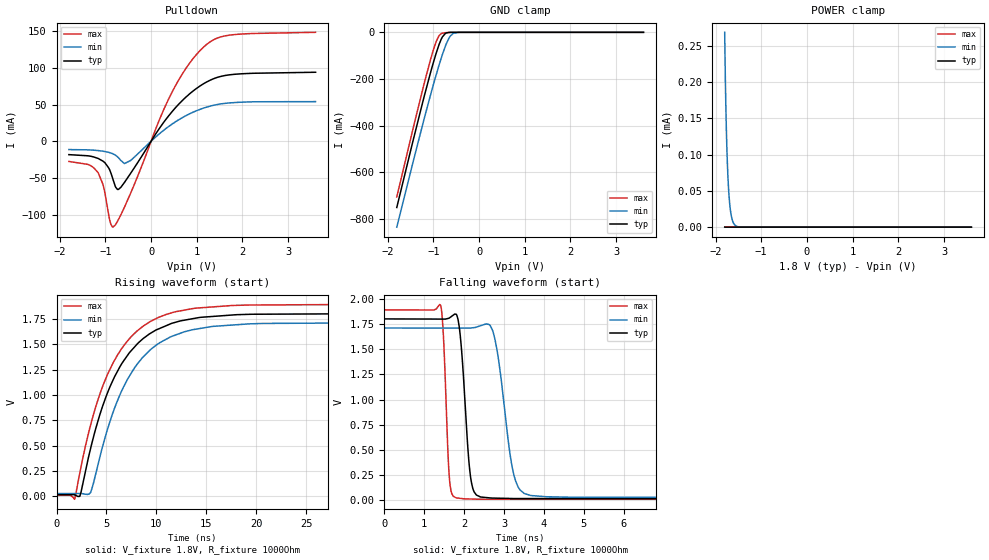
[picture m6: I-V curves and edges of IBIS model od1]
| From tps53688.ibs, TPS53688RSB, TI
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|   od1 Model
[Model]   od1
Model_type   Open_drain
Polarity   Non-Inverting
Vmeas = 0.9
Vref = 1.8
Cref = 2pF
Rref = 1000
|   typ   min   max
C_comp   1.818pF   1.802pF   1.852pF
[Voltage Range]   1.8   1.71   1.89
|Junction Temperature
[Temperature Range]   25   125   -40
[Pullup Reference]   1.8   1.71   1.89
[Pulldown Reference]   0   0   0
[Power Clamp Reference]   1.8   1.71   1.89
[GND Clamp Reference]   0   0   0
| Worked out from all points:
|   slope of the pulldown table from 0 to 0.27 V, typ, clamps not added: 10.7 ohm
|   GND clamp passes 1 mA (typ) near -0.67 V on its own axis
|   falling waveform, V_fixture 1.8V, R_fixture 1000Ohm: 20-80 % time 177ps typ, 319ps min, 110ps max; typ from 1.8 V to 0.018 V
|   rising waveform, V_fixture 1.8V, R_fixture 1000Ohm: 20-80 % time 4.38ns typ, 4.39ns min, 4.31ns max; typ from 0.018 V to 1.8 V
[Pulldown]
|   Voltage   I(typ)   I(min)   I(max)
-1.8V     -18.28mA   -11.37mA   -27.6mA
-1.163V   -23.4mA    -12.72mA   -42.59mA
-1.055V   -27.13mA   -13.6mA    -58.57mA
-903.6mV  -39.52mA   -15.62mA   -108mA
-838.8mV  -51.1mA    -17.06mA   -117.1mA
-736.2mV  -65.68mA   -21.17mA   -109.2mA
-660.6mV  -62.69mA   -26.31mA   -100.2mA
-444.6mV  -43.43mA   -26.16mA   -70.28mA
462.6mV   40.55mA    23.51mA    67.36mA
1.143V    78.14mA    45.04mA    128mA
1.721V    90.51mA    52.22mA    144.6mA
3.6V      93.99mA    53.98mA    148.4mA
[GND Clamp]
|   Voltage   I(typ)   I(min)   I(max)
-1.8V     -751mA     -835.3mA   -705.6mA
-1.217V   -287.5mA   -382.9mA   -231.9mA
-1.055V   -168.1mA   -263.9mA   -112.3mA
-990mV    -123.4mA   -218.2mA   -69.83mA
-930.6mV  -85.17mA   -177.5mA   -36.7mA
-882mV    -56.7mA    -145.4mA   -16.96mA
-801mV    -19.58mA   -95.08mA   -3.736mA
-736.2mV  -4.621mA   -59.16mA   -1.662mA
-660.6mV  -580.1uA   -25.84mA   -535.1uA
-563.4mV  -53.04uA   -4.177mA   -64.9uA
-390.6mV  -457.9nA   -36.71uA   -236.7nA
3.6V      0A         0A         0A
[POWER Clamp]
|   Voltage   I(typ)   I(min)   I(max)
-1.8V     119.9nA    268.6uA    121.8pA
-1.795V   90.19nA    242.7uA    60.9pA
-1.784V   60.2nA     198uA      0A
-1.773V   39.27nA    161.5uA    0A
-1.762V   24.3nA     131.5uA    0A
-1.741V   6.328nA    86.89uA    0A
-1.719V   0A         56.99uA    0A
-1.692V   0A         33.25uA    0A
-1.66V    0A         17.1uA     0A
-1.616V   0A         6.839uA    0A
-1.562V   0A         2.059uA    0A
3.6V      0A         0A         0A
[Ramp]
R_load = 1000
|   typ   min   max
dV/dt_r   1.06947/4.36309e-09   1.0088/4.39564e-09   1.12741/4.31284e-09
dV/dt_f   1.06947/1.77224e-10   1.0088/3.18056e-10   1.12741/1.09567e-10
[Falling Waveform]
V_fixture = 1.8V
V_fixture_min = 1.71V
V_fixture_max = 1.89V
R_fixture = 1000Ohm
C_fixture = 0F
|   Time   V(typ)   V(min)   V(max)
0s        1.8V       1.71V      1.89V
1.406ns   1.798V     1.709V     1.939V
1.633ns   1.811V     1.709V     203.1mV
1.816ns   1.836V     1.709V     24.69mV
2.156ns   243.7mV    1.709V     14.3mV
2.367ns   42.31mV    1.727V     11.94mV
2.77ns    22.92mV    1.601V     11.94mV
3.373ns   18.68mV    119.9mV    11.94mV
4.88ns    18.67mV    30.36mV    11.94mV
500ns     17.56mV    28.66mV    10.99mV
[Rising Waveform]
V_fixture = 1.8V
V_fixture_min = 1.71V
V_fixture_max = 1.89V
R_fixture = 1000Ohm
C_fixture = 0F
|   Time   V(typ)   V(min)   V(max)
0s        17.56mV    28.66mV    10.99mV
1.82ns    15.58mV    29.05mV    -25.48mV
2.345ns   4.669mV    29.16mV    237.4mV
3.403ns   468.5mV    37.67mV    698.9mV
5.381ns   1.086V     745.9mV    1.257V
7.509ns   1.438V     1.218V     1.576V
9.421ns   1.607V     1.446V     1.724V
11.44ns   1.7V       1.572V     1.805V
17.63ns   1.787V     1.688V     1.881V
500ns     1.8V       1.71V      1.89V
